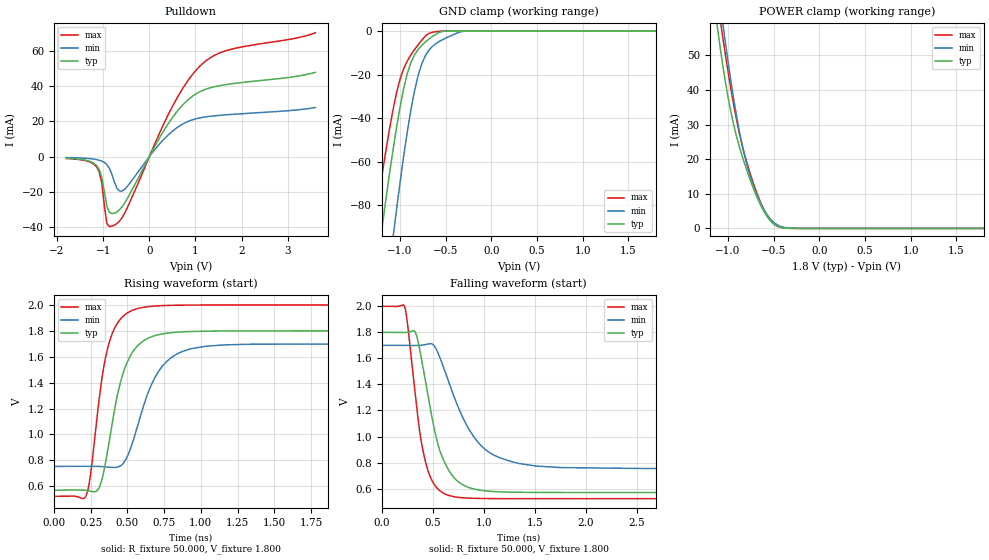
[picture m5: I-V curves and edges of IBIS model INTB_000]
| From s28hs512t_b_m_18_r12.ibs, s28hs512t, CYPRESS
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|   Model INTB_000
[Model] INTB_000
Model_type Open_drain
Polarity   Inverting
Enable   Active-High
Vmeas =  0.900V
Cref =   15.0000pF
Rref =   6.2000k
Vref =   1.8000V
C_comp   5.334pF   5.23pF   5.767pF
[Temperature Range]   25.000   0.125k   -40.000
[Voltage Range]   1.800V   1.700V   2.000V
[Pullup Reference]   1.800V   1.700V   2.000V
[Pulldown Reference]   0.0V   0.0V   0.0V
[POWER Clamp Reference]   1.800V   1.700V   2.000V
[GND Clamp Reference]   0.0V   0.0V   0.0V
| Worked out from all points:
|   slope of the pulldown table from 0 to 0.27 V, typ, clamps not added: 21 ohm
|   GND clamp passes 1 mA (typ) near -0.59 V on its own axis
|   POWER clamp passes 1 mA (typ) near -0.48 V on its own axis
|   rising waveform, R_fixture 50.000, V_fixture 1.800: 20-80 % time 141ps typ, 191ps min, 112ps max; typ from 0.57 V to 1.8 V
|   falling waveform, R_fixture 50.000, V_fixture 1.800: 20-80 % time 209ps typ, 344ps min, 149ps max; typ from 1.8 V to 0.57 V
[Pulldown]
|Voltage   I(typ)   I(min)   I(max)
-1.8V     -919.4uA   -496.1uA   -1.054mA
-1.14V    -5.184mA   -1.692mA   -5.957mA
-1.03V    -11.81mA   -2.55mA    -15.02mA
-920mV    -28.09mA   -4.545mA   -38.04mA
-755mV    -32.07mA   -14.63mA   -38.83mA
-645mV    -30.07mA   -19.53mA   -36.53mA
-535mV    -26.34mA   -18.54mA   -32.06mA
455mV     20.46mA    13.41mA    26.17mA
785mV     30.97mA    19.33mA    41.2mA
1.115V    37.1mA     22.09mA    51.84mA
1.72V     41.1mA     23.84mA    60.55mA
3.6V      47.81mA    27.87mA    70.26mA
[GND_clamp]
|Voltage   I(typ)   I(min)   I(max)
-1.8V     -294mA     -373mA     -247.3mA
-1.28V    -116.8mA   -168.5mA   -89.46mA
-1.2V     -91.34mA   -138.7mA   -67.04mA
-1.08V    -55.6mA    -96.11mA   -36.91mA
-1.04V    -44.83mA   -82.66mA   -28.74mA
-1V       -34.98mA   -69.76mA   -22.14mA
-920mV    -19.48mA   -46.23mA   -13.73mA
-800mV    -8.377mA   -20.18mA   -6.205mA
-680mV    -3.579mA   -8.59mA    -1.029mA
-560mV    -408.3uA   -4.544mA   -113.8uA
-280mV    -162.8nA   -73.51uA   -82.13nA
1.8V      272.8pA    325nA      188.3pA
[POWER_clamp]
|Voltage   I(typ)   I(min)   I(max)
-1.8V     236.7mA    239.1mA    251.1mA
-1.123V   59.68mA    73.25mA    67.66mA
-1.086V   52.46mA    65.42mA    60.6mA
-1.049V   45.83mA    57.89mA    53.9mA
-938mV    30.03mA    37.57mA    35.87mA
-864mV    22.62mA    26.6mA     26.18mA
-790mV    16.52mA    18.14mA    18.76mA
-716mV    11.21mA    11.92mA    12.63mA
-642mV    6.708mA    7.258mA    7.47mA
-494mV    1.178mA    1.619mA    1.205mA
-272mV    6.291uA    28.11uA    4.439uA
1.8V      0A         0A         0A
[Ramp]
| variable   typ   min   max
dV/dt_r   0.676/0.206n   0.568/0.300n   0.817/0.151n
dV/dt_f   0.738/0.209n   0.568/0.344n   0.887/0.149n
R_load = 50.000
[Rising Waveform]
R_fixture= 50.000
V_fixture= 1.800
V_fixture_min= 1.700
V_fixture_max= 2.000
|time   V(typ)   V(min)   V(max)
0s        570mV      753.8mV    522.4mV
218ps     568.7mV    754.6mV    524.5mV
251ps     561.4mV    754.5mV    700.4mV
308ps     588.6mV    753.2mV    1.272V
409ps     1.167V     745.3mV    1.811V
487ps     1.525V     802.4mV    1.928V
582ps     1.698V     1.115V     1.975V
738ps     1.776V     1.527V     1.995V
1.032ns   1.797V     1.681V     1.999V
6ns       1.8V       1.7V       2V
[Falling Waveform]
R_fixture= 50.000
V_fixture= 1.800
V_fixture_min= 1.700
V_fixture_max= 2.000
|time   V(typ)   V(min)   V(max)
0s        1.8V       1.7V       2V
224ps     1.799V     1.7V       1.998V
328ps     1.801V     1.699V     1.327V
380ps     1.636V     1.7V       996.1mV
452ps     1.323V     1.71V      739.5mV
551ps     939.2mV    1.643V     596.6mV
661ps     733.9mV    1.409V     546.9mV
967ps     587.2mV    935.3mV    524.2mV
1.343ns   571.7mV    792.9mV    522.6mV
6ns       570mV      753.8mV    522.4mV
